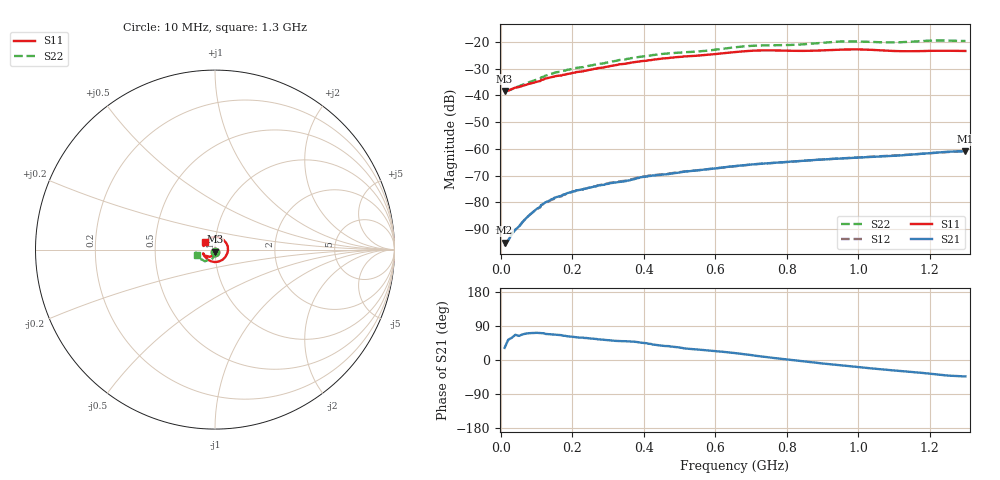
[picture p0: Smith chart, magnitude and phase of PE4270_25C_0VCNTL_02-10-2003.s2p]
!Peregrine Semiconductor Corp.
!S-Parameter Data for Device PE4248 in ISO PATH with TEMP = 25C
!File Created On: 02-10-2003
!Start Frequency = 1.000E+01
!Stop Frequency = 1.300E+03
!Number of Points = 145
# MHZ S DB R 75
!Freq  S11MAG  S11PH  S12MAG  S12PH  S21MAG  S21PH  S22MAG  S22PH
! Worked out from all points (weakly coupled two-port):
!   145 points, 10 MHz to 1.3 GHz, reference 75 ohm
!   highest |S21| = -60.85 dB at 1.3 GHz (marker M1); lowest = -95.2 dB at 10 MHz (marker M2)
!   lowest |S11| = -38.3 dB at 10 MHz (marker M3), VSWR 1.02, Z = 75.1 - j1.82 ohm
!   |S11| at or under -10 dB: start of sweep to end of sweep
!   |S22| runs from -38.3 to -19.4 dB; largest |S21 - S12| = 0.00053
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10  -38.31 -87.1  -95.16 32.0  -96.46 22.3  -38.34 -87.1
20  -38.18 -85.1  -94.32 53.3  -94.32 50.6  -38.24 -85.6
130  -33.53 -93.2  -79.73 68.5  -79.93 72.1  -32.39 -87.7
150  -32.83 -95.0  -78.26 66.8  -78.42 71.2  -31.44 -88.3
170  -32.51 -96.1  -77.55 65.5  -77.75 70.2  -31.05 -88.8
184  -32.02 -97.6  -76.64 62.9  -76.70 68.2  -30.45 -89.3
230  -30.97 -102.3  -75.18 59.0  -75.19 65.5  -29.38 -92.4
304  -29.04 -111.9  -72.91 52.0  -72.73 60.6  -27.49 -100.3
440  -26.37 -125.3  -69.81 38.9  -69.66 49.9  -24.65 -109.5
568  -24.92 -139.9  -67.78 26.2  -67.75 40.5  -23.36 -121.4
664  -23.65 -149.4  -66.33 17.2  -66.39 34.0  -21.83 -128.9
736  -23.12 -153.4  -65.52 8.5  -65.52 27.4  -21.26 -131.7
832  -23.31 -162.7  -64.61 -1.9  -64.62 19.9  -20.97 -140.7
880  -23.23 -109.4  -64.15 -7.0  -64.15 16.5  -20.49 -145.3
904  -23.10 -72.7  -63.95 -9.6  -63.97 14.6  -20.21 -146.9
940  -22.90 -16.5  -63.69 -13.0  -63.65 12.0  -19.87 -148.3
1000  -22.76 18.8  -63.23 -18.7  -63.21 7.5  -19.80 -150.3
1048  -23.00 89.0  -62.93 -23.1  -62.88 4.1  -20.03 -154.2
1096  -23.33 146.8  -62.63 -27.2  -62.54 1.1  -20.13 -160.1
1120  -23.42 162.8  -62.45 -29.1  -62.36 -0.3  -20.06 -163.2
1216  -23.28 148.9  -61.45 -37.6  -61.47 -5.9  -19.43 -170.7
1300  -23.35 142.8  -60.85 -43.4  -60.90 -9.6  -19.61 -163.5
